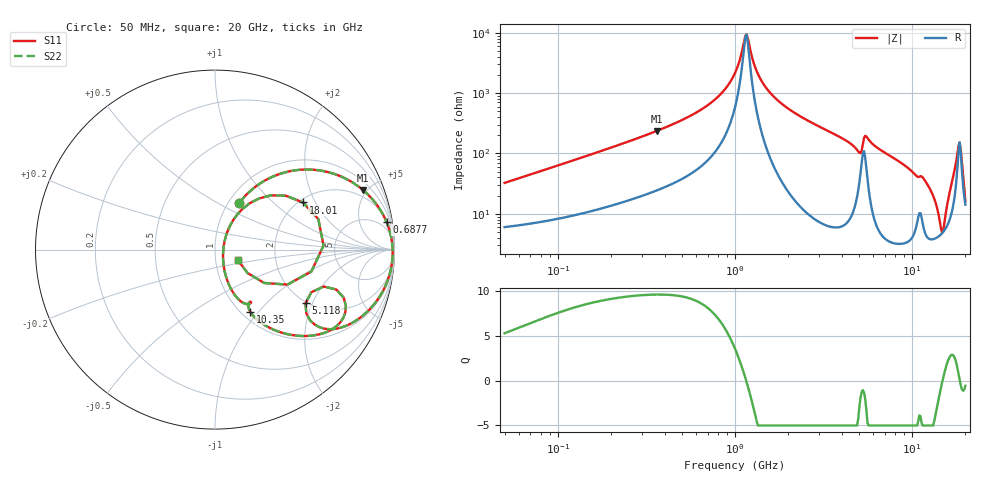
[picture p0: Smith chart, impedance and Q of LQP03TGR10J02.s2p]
!Murata Part Number: LQP03TGR10J02
!These Parameters are Measured in Series Mode Connection
!  o--[Z]--o
!Port1  Port2
!  o-------o
!Freq. Start=50[MHz] Stop=20[GHz], 401[Steps]
# Hz S RI R 50
!Freq.(Hz) S11(Real) S11(Imag) S21(Real) S21(Imag) S12(Real) S12(Imag) S22(Real) S22(Imag)
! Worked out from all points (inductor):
!   401 points, 50 MHz to 20 GHz, reference 50 ohm
!   read as one part in series: L = 101 nH near 51.52 MHz
!   highest Q = 9.63 at 361.1 MHz (marker M1), where L = 103 nH
!   self-resonance near 1.144 GHz
!   S11 on the Smith chart (normalised r, x): 50 MHz: 1.12, +0.64; 687.7 MHz: 2, +12; 5.118 GHz: 1.96, -1.79; 10.35 GHz: 1.10, -0.90; 18.01 GHz: 2.10, +1.60; 20 GHz: 1.28, -0.16
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5e7  0.1354 0.2606  0.8646 -0.2606  0.8646 -0.2606  0.1354 0.2606
1.364002e8  0.4314 0.4394  0.5686 -0.4394  0.5686 -0.4394  0.4314 0.4394
3.611186e8  0.8235 0.3328  0.1765 -0.3328  0.1765 -0.3328  0.8235 0.3328
3.721004e8  0.8323 0.3253  0.1677 -0.3253  0.1677 -0.3253  0.8323 0.3253
6.87656e8  0.9558 0.1537  0.0442 -0.1537  0.0442 -0.1537  0.9558 0.1537
8.608917e8  0.9774 0.0878  0.0226 -0.0878  0.0226 -0.0878  0.9774 0.0878
1e9  0.9857 0.0435  0.0143 -0.0435  0.0143 -0.0435  0.9857 0.0435
1.161586e9  0.9895 -0.00124  0.0105 0.00124  0.0105 0.00124  0.9895 -0.00124
1.329223e9  0.989 -0.0422  0.011 0.0422  0.011 0.0422  0.989 -0.0422
1.521052e9  0.9845 -0.0841  0.0155 0.0841  0.0155 0.0841  0.9845 -0.0841
2.728004e9  0.9052 -0.2796  0.0948 0.2796  0.0948 0.2796  0.9052 -0.2796
4.539627e9  0.66 -0.4426  0.34 0.4426  0.34 0.4426  0.66 -0.4426
5.117541e9  0.5044 -0.2994  0.4956 0.2994  0.4956 0.2994  0.5044 -0.2994
5.598765e9  0.7256 -0.3524  0.2744 0.3524  0.2744 0.3524  0.7256 -0.3524
7.442007e9  0.4639 -0.4804  0.5361 0.4804  0.5361 0.4804  0.4639 -0.4804
1.034674e10  0.1962 -0.3457  0.8038 0.3457  0.8038 0.3457  0.1962 -0.3457
1.257102e10  0.0937 -0.2272  0.9063 0.2272  0.9063 0.2272  0.0937 -0.2272
1.482269e10  0.046 -0.00352  0.954 0.00352  0.954 0.00352  0.046 -0.00352
1.670968e10  0.1544 0.2276  0.8456 -0.2276  0.8456 -0.2276  0.1544 0.2276
1.800918e10  0.4896 0.263  0.5104 -0.263  0.5104 -0.263  0.4896 0.263
1.88369e10  0.5368 -0.1226  0.4632 0.1226  0.4632 0.1226  0.5368 -0.1226
2e10  0.1283 -0.0607  0.8717 0.0607  0.8717 0.0607  0.1283 -0.0607
